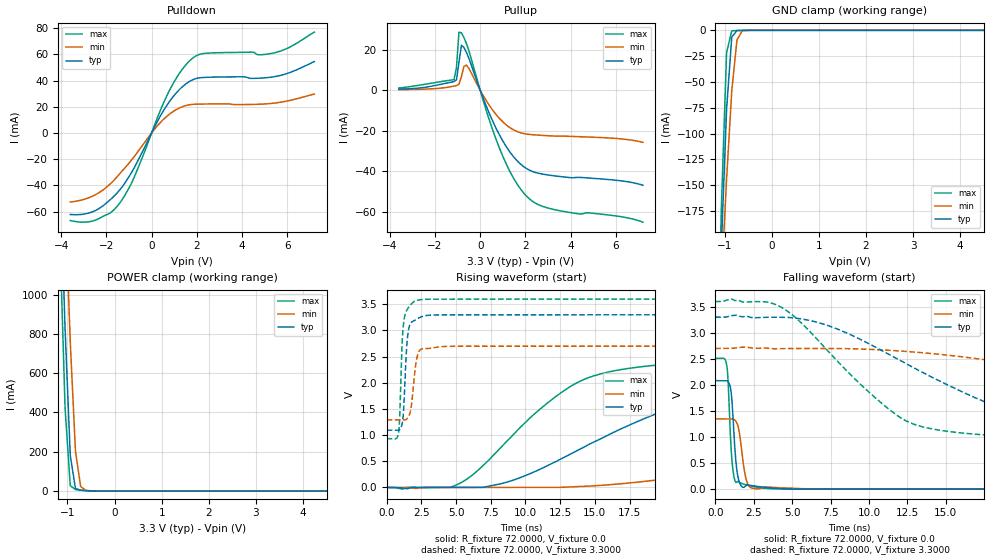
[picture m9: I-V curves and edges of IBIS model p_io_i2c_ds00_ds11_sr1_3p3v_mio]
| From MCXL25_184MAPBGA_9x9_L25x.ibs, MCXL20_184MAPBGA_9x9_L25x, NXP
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[Model] p_io_i2c_ds00_ds11_sr1_3p3v_mio
|   Model p_io_i2c_ds00_ds11_sr1_3p3v_mio
| This model was characterised for following simulation conditions:
| External (pad) voltage:
|   - Typ: 3.3V,   - Min: 2.7V,   - Max: 3.6V
| Library cells for typ/min/max conditions are connected as defined below:
|  pad - External Pad
|  ipp_do_lv - Core Input
|  ipp_obe_lv - Output Buffer Enable
|  IOGC - NC
|  REFH3V3 - REFH3V3
|  REFL3V3 - REFL3V3
|  ZI - NC
|  abut_ncal_vddio[1] - vddio
|  abut_ncal_vddio[2] - vddio
|  abut_ncal_vddio[3] - vssio
|  abut_ncal_vddio[4] - vddio
|  abut_ncal_vddio[5] - vddio
|  abut_ncal_vddio[6] - vssio
|  abut_pcal_vddio[1] - vssio
|  abut_pcal_vddio[2] - vssio
|  abut_pcal_vddio[3] - vddio
|  abut_pcal_vddio[4] - vssio
|  abut_pcal_vddio[5] - vssio
|  abut_pcal_vddio[6] - vddio
|  ipp_do_1p8v - ipp_do_1p8v
|  ipp_dse_lv[0] - 0
|  ipp_dse_lv[1] - vdd_lv
|  ipp_eftd_lv - NC
|  ipp_ina_mux_vddio - NC
|  ipp_ina_mux_vddio[0] - NC
|  ipp_ina_mux_vddio[1] - NC
|  ipp_ina_r0_vddio - NC
|  ipp_ina_r0a_vddio - NC
|  ipp_ina_r0b_vddio - NC
|  ipp_ina_r0c_vddio - NC
|  ipp_ina_r0d_vddio - NC
|  ipp_ina_r0e_vddio - NC
|  ipp_ina_r0f_vddio - NC
|  ipp_ina_r300_vddio - NC
|  ipp_ina_r300a_vddio - NC
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Model_type I/O
Polarity   Non-Inverting
Enable   Active-High
Vinl =   0.9900V
Vinh =   2.3100V
Vmeas =  1.6500V
Cref =   30.0000pF
Rref =   1.0000M
Vref =   3.3000V
C_comp   1.4149pF   1.3702pF   1.4746pF
|C_comp_pullup   0.5856pF   0.6310pF   0.5569pF
|C_comp_pulldown   0.7314pF   0.7413pF   0.7169pF
[Model Spec]
| variable   typ   min   max
Vinh   2.3100V   1.8900V   2.5200V
Vinl   0.9900V   0.8100V   1.0800V
[Temperature Range]   25.0000   0.1250k   -40.0000
[Voltage Range]   3.3000V   2.7000V   3.6000V
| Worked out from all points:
|   slope of the pulldown table from 0 to 0.495 V, typ, clamps not added: 30.7 ohm
|   slope of the pullup table from 0 to 0.495 V, typ, clamps not added: 35.9 ohm
|   GND clamp passes 1 mA (typ) near -0.75 V on its own axis
|   POWER clamp passes 1 mA (typ) near -0.57 V on its own axis
|   rising waveform, R_fixture 72.0000, V_fixture 0.0: 20-80 % time 10.9ns typ, 23.5ns min, 6.49ns max; typ from 0 V to 2.08 V
|   rising waveform, R_fixture 72.0000, V_fixture 3.3000: 20-80 % time 264ps typ, 350ps min, 236ps max; typ from 1.09 V to 3.3 V
|   falling waveform, R_fixture 72.0000, V_fixture 0.0: 20-80 % time 290ps typ, 376ps min, 254ps max; typ from 2.08 V to 0 V
|   falling waveform, R_fixture 72.0000, V_fixture 3.3000: 20-80 % time 9.26ns typ, 20.2ns min, 5.58ns max; typ from 3.3 V to 1.09 V
[Pulldown]
|Voltage   I(typ)   I(min)   I(max)
-3.6V     -62.23mA   -52.7mA    -66.82mA
-2.5V     -59.31mA   -47.25mA   -66.6mA
-1.84V    -51.07mA   -39.04mA   -61.22mA
-1.4V     -43.29mA   -30.9mA    -53.31mA
-850mV    -29.1mA    -19.8mA    -36.9mA
140mV     4.939mA    3.095mA    6.557mA
800mV     24.23mA    14.5mA     32.79mA
1.35V     35.15mA    20.01mA    48.49mA
1.79V     40.41mA    21.82mA    56.77mA
2.45V     42.54mA    22.16mA    60.95mA
5.42V     42.98mA    22.81mA    61.18mA
7.2V      54.57mA    29.73mA    77.07mA
[Pullup]
|Voltage   I(typ)   I(min)   I(max)
-3.6V     528.7uA    283.5uA    1.096mA
-1.16V    4.253mA    2.05mA     5.214mA
-1.05V    5.16mA     2.299mA    11.28mA
-940mV    13.88mA    2.903mA    28.69mA
-830mV    22.22mA    6.81mA     28.28mA
-720mV    21.08mA    11.76mA    25.94mA
-610mV    18.66mA    12.39mA    23.05mA
820mV     -21.34mA   -13.5mA    -27.66mA
1.48V     -32.86mA   -19.56mA   -43.47mA
2.03V     -38.49mA   -21.57mA   -52mA
3.24V     -42.16mA   -22.57mA   -58.77mA
7.2V      -46.85mA   -25.7mA    -65.08mA
[GND_clamp]
|Voltage   I(typ)   I(min)   I(max)
-3.6V     -4.327A    -3.181A    -5.901A
-1.18V    -358.9mA   -350.6mA   -379.3mA
-1.07V    -208.2mA   -244.2mA   -170.8mA
-960mV    -76.59mA   -144.3mA   -21.58mA
-850mV    -6.561mA   -58.74mA   -508.1uA
-740mV    -273.3uA   -9.382mA   -183.5uA
-630mV    -73.8uA    -593.1uA   -76.7uA
-410mV    -3.432uA   -9.016uA   -2.096uA
7.2V      0A         0A         0A
[POWER_clamp]
|Voltage   I(typ)   I(min)   I(max)
-3.6V     20.44A     18.76A     22.48A
-1.16V    1.647A     2.216A     1.289A
-1.05V    823.6mA    1.482A     419.2mA
-940mV    180.4mA    758.9mA    26.72mA
-830mV    12.56mA    202.9mA    6.794mA
-720mV    3.422mA    22.23mA    3.58mA
-610mV    1.373mA    2.923mA    1.344mA
7.2V      0A         0A         0A
[Ramp]
| variable   typ   min   max
dV/dt_r  1.2490/10.9328n   0.8052/23.4542n   1.5058/6.4834n
dV/dt_f  1.3238/9.2573n   0.8433/20.2060n   1.6012/5.5813n
R_load = 72.0000
[Rising Waveform]
R_fixture= 72.0000
V_fixture= 0.0
V_fixture_min= 0.0
V_fixture_max= 0.0
|time   V(typ)   V(min)   V(max)
0s        1.645nV    121.1nV    5.564nV
4.722ns   -107uV     -493.5uV   12.4mV
8.651ns   99.94mV    -27.76uV   881.4mV
11.33ns   382.1mV    408.2uV    1.559V
14.02ns   745.3mV    17.94mV    2.041V
21.02ns   1.559V     194.9mV    2.372V
31ns      1.917V     595.2mV    2.468V
41.94ns   2.015V     981.2mV    2.496V
52.23ns   2.051V     1.151V     2.505V
131.4ns   2.082V     1.342V     2.51V
[Rising Waveform]
R_fixture= 72.0000
V_fixture= 3.3000
V_fixture_min= 2.7000
V_fixture_max= 3.6000
|time   V(typ)   V(min)   V(max)
0s        1.093V     1.29V      931.4mV
861.3ps   1.093V     1.29V      1.053V
939.5ps   1.104V     1.29V      1.34V
1.124ns   1.226V     1.29V      2.807V
1.321ns   2.045V     1.292V     3.297V
1.453ns   2.723V     1.309V     3.387V
1.629ns   3.075V     1.385V     3.459V
2.176ns   3.217V     2.472V     3.574V
2.603ns   3.271V     2.652V     3.592V
131.4ns   3.3V       2.7V       3.6V
[Falling Waveform]
R_fixture= 72.0000
V_fixture= 0.0
V_fixture_min= 0.0
V_fixture_max= 0.0
|time   V(typ)   V(min)   V(max)
0s        2.082V     1.348V     2.51V
749.7ps   2.081V     1.348V     2.37V
834ps     2.064V     1.348V     2.077V
1.043ns   1.835V     1.35V      722.8mV
1.296ns   694.9mV    1.318V     152.5mV
1.588ns   118.1mV    1.048V     128.9mV
1.88ns    39.76mV    380.4mV    93.16mV
2.114ns   82.19mV    99.92mV    75.03mV
3.332ns   30.82mV    43.2mV     14.05mV
131.4ns   166.7nV    3.504uV    20.79nV
[Falling Waveform]
R_fixture= 72.0000
V_fixture= 3.3000
V_fixture_min= 2.7000
V_fixture_max= 3.6000
|time   V(typ)   V(min)   V(max)
0s        3.3V       2.7V       3.6V
3.946ns   3.299V     2.693V     3.54V
7.117ns   3.161V     2.699V     2.719V
12.3ns    2.425V     2.645V     1.328V
17.7ns    1.656V     2.478V     1.038V
20.46ns   1.413V     2.359V     997.6mV
25.7ns    1.253V     2.111V     962mV
36.06ns   1.152V     1.66V      940mV
46.06ns   1.12V      1.475V     934.4mV
131.4ns   1.094V     1.295V     931.4mV
